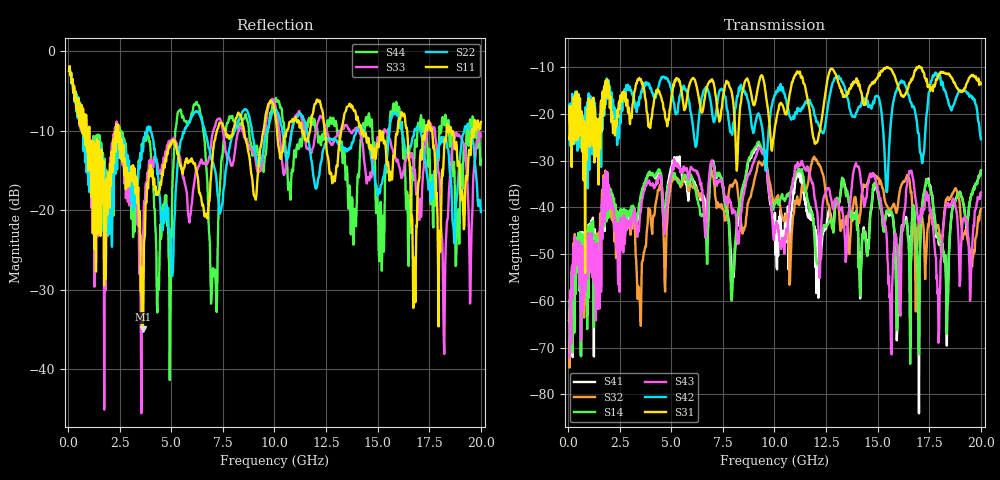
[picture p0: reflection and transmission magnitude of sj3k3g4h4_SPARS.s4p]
! FILE: E:\users\goganessyan\GBX_Backplane\FR408_backplane\1m_OUTBOUND_NEXT\sj3k3g4h4_SPARS.s4p
# MHZ S RI R 50.00
! FREQ  S11  S12  S13  S14
!  S21  S22  S23  S24
!  S31  S32  S33  S34
!  S41  S42  S43  S44
!  REAL  IMAG  REAL  IMAG  REAL  IMAG  REAL  IMAG
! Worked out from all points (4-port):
!   799 points, 50 MHz to 20 GHz, reference 50 ohm
!   strongest paths, dB at 50 MHz, 5.025 GHz, 10.03 GHz, 15.03 GHz, 20 GHz:
!     S31: -18.5, -15.8, -22.6, -12.1, -13.6
!     S42: -18.1, -15.5, -15.9, -16.3, -25.4
!     S43: -72.1, -32.7, -44.4, -36.6, -36.8
!     S14: -69.3, -33.5, -38.8, -37.3, -32.2
!     S32: -62.4, -34.5, -38.5, -34.0, -40.4
!     S41: -64.2, -31.5, -41.2, -37.0, -32.2
!   lowest |S11| = -35.0 dB at 3.625 GHz (marker M1), VSWR 1.04, Z = 48.8 - j1.31 ohm
!   |S11| at or under -10 dB: 1.027 GHz to 2.325 GHz (1.298 GHz wide, 77.4 % of centre); 2.436 GHz to 7.21 GHz (4.774 GHz wide, 99 % of centre); 18.56 GHz to 19.56 GHz (997.7 MHz wide, 5.23 % of centre)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
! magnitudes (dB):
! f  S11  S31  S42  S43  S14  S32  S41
! 50 MHz  -2.5  -18.5  -18.1  -72.1  -69.3  -62.4  -64.2
! 1.8 GHz  -17.5  -14.4  -13.1  -32.9  -35.8  -32.1  -34.9
! 2.9 GHz  -16.6  -19.8  -13.8  -42.8  -41.7  -43.7  -42.3
! 3.625 GHz  -35.0  -13.9  -13.9  -37.6  -35.8  -51.3  -36.0
! 14.88 GHz  -12.9  -13.0  -16.3  -33.6  -34.8  -33.2  -34.7
! 15.95 GHz  -10.4  -13.6  -14.5  -48.1  -66.2  -40.6  -65.6
! 20 GHz  -8.9  -13.6  -25.4  -36.8  -32.2  -40.4  -32.2
